DATA_BLOCK "PR"
TITLE =
VERSION : 0.1


  STRUCT
   rKmA_DlmHzl : INT ;	//EVS 100 HIZLI DOLUM % HIZ SET DEGERI
   rKmA_DlmYvs : INT ;	//EVS 100 YAVAS DOLUM % HIZ SET DEGERI
   rKmA_BsltHzl : INT ;	//EVS 100 HIZLI DOLUM % HIZ SET DEGERI
   rKmA_BsltYvs : INT ;	//EVS 100 YAVAS DOLUM % HIZ SET DEGERI
   rKmB_DlmHzl : INT ;	//EVS 100 HIZLI DOLUM % HIZ SET DEGERI
   rKmB_DlmYvs : INT ;	//EVS 100 YAVAS DOLUM % HIZ SET DEGERI
   rKmB_BsltHzl : INT ;	//EVS 100 HIZLI DOLUM % HIZ SET DEGERI
   rKmB_BsltYvs : INT ;	//EVS 100 YAVAS DOLUM % HIZ SET DEGERI
   rSd_BsltHzl : INT ;	//EVS 100 HIZLI DOLUM % HIZ SET DEGERI
   rSd_BsltYvs : INT ;	//EVS 100 YAVAS DOLUM % HIZ SET DEGERI
   rKl_BsltHzl : INT ;	//EVS 100 HIZLI DOLUM % HIZ SET DEGERI
   rKl_BsltYvs : INT ;	//EVS 100 YAVAS DOLUM % HIZ SET DEGERI
   rFl_BsltHzl : INT ;	//EVS 100 HIZLI DOLUM % HIZ SET DEGERI
   rFl_BsltYvs : INT ;	//EVS 100 YAVAS DOLUM % HIZ SET DEGERI
   rSl_BsltHzl : INT ;	//EVS 100 HIZLI DOLUM % HIZ SET DEGERI
   rSl_BsltYvs : INT ;	//EVS 100 YAVAS DOLUM % HIZ SET DEGERI
   rHm_BsltHzl : INT ;	//EVS 100 HIZLI DOLUM % HIZ SET DEGERI
   rHm_BsltYvs : INT ;	//EVS 100 YAVAS DOLUM % HIZ SET DEGERI
   rAn_BsltHzl : INT ;	//EVS 100 HIZLI DOLUM % HIZ SET DEGERI
   rAn_BsltYvs : INT ;	//EVS 100 YAVAS DOLUM % HIZ SET DEGERI
   YD : INT ;
   YD1 : INT ;
   YD2 : INT ;
   YD3 : INT ;
   YD4 : INT ;
   wKmA_DlmHzl { S7_m_c := 'true' }: INT ;	//EVS 100 HIZLI DOLUM % HIZ SET DEGERI
   wKmA_DlmYvs { S7_m_c := 'true' }: INT ;	//EVS 100 YAVAS DOLUM % HIZ SET DEGERI
   wKmA_BsltHzl { S7_m_c := 'true' }: INT ;	//EVS 100 HIZLI DOLUM % HIZ SET DEGERI
   wKmA_BsltYvs { S7_m_c := 'true' }: INT ;	//EVS 100 YAVAS DOLUM % HIZ SET DEGERI
   wKmB_DlmHzl { S7_m_c := 'true' }: INT ;	//EVS 100 HIZLI DOLUM % HIZ SET DEGERI
   wKmB_DlmYvs { S7_m_c := 'true' }: INT ;	//EVS 100 YAVAS DOLUM % HIZ SET DEGERI
   wKmB_BsltHzl { S7_m_c := 'true' }: INT ;	//EVS 100 HIZLI DOLUM % HIZ SET DEGERI
   wKmB_BsltYvs { S7_m_c := 'true' }: INT ;	//EVS 100 YAVAS DOLUM % HIZ SET DEGERI
   wSd_BsltHzl { S7_m_c := 'true' }: INT ;	//EVS 100 HIZLI DOLUM % HIZ SET DEGERI
   wSd_BsltYvs { S7_m_c := 'true' }: INT ;	//EVS 100 YAVAS DOLUM % HIZ SET DEGERI
   wKl_BsltHzl { S7_m_c := 'true' }: INT ;	//EVS 100 HIZLI DOLUM % HIZ SET DEGERI
   wKl_BsltYvs { S7_m_c := 'true' }: INT ;	//EVS 100 YAVAS DOLUM % HIZ SET DEGERI
   wFl_BsltHzl { S7_m_c := 'true' }: INT ;	//EVS 100 HIZLI DOLUM % HIZ SET DEGERI
   wFl_BsltYvs { S7_m_c := 'true' }: INT ;	//EVS 100 YAVAS DOLUM % HIZ SET DEGERI
   wSl_BsltHzl { S7_m_c := 'true' }: INT ;	//EVS 100 HIZLI DOLUM % HIZ SET DEGERI
   wSl_BsltYvs { S7_m_c := 'true' }: INT ;	//EVS 100 YAVAS DOLUM % HIZ SET DEGERI
   wHm_BsltHzl { S7_m_c := 'true' }: INT ;	//EVS 100 HIZLI DOLUM % HIZ SET DEGERI
   wHm_BsltYvs { S7_m_c := 'true' }: INT ;	//EVS 100 YAVAS DOLUM % HIZ SET DEGERI
   wAn_BsltHzl { S7_m_c := 'true' }: INT ;	//EVS 100 HIZLI DOLUM % HIZ SET DEGERI
   wAn_BsltYvs { S7_m_c := 'true' }: INT ;	//EVS 100 YAVAS DOLUM % HIZ SET DEGERI
   YD5 : INT ;
   KmANEM_ORAN { S7_m_c := 'true' }: REAL ;	//NEM ORAN
   KmBNEM_ORAN { S7_m_c := 'true' }: REAL ;	//NEM ORAN
   SdNEM_ORAN { S7_m_c := 'true' }: REAL ;	//NEM ORAN
   DlNEM_ORAN { S7_m_c := 'true' }: REAL ;	//NEM ORAN
   KlNEM_ORAN { S7_m_c := 'true' }: REAL ;	//NEM ORAN
   FlNEM_ORAN { S7_m_c := 'true' }: REAL ;	//NEM ORAN
   SlNEM_ORAN { S7_m_c := 'true' }: REAL ;	//NEM ORAN
   HmNEM_ORAN { S7_m_c := 'true' }: REAL ;	//NEM ORAN
   AnNEM_ORAN { S7_m_c := 'true' }: REAL ;	//NEM ORAN
   Renk1NEM_ORAN : REAL ;	//NEM ORAN
   Renk2NEM_ORAN : REAL ;	//NEM ORAN
   Renk3NEM_ORAN : REAL ;	//NEM ORAN
   Renk4NEM_ORAN : REAL ;	//NEM ORAN
   KmA_TolKg { S7_m_c := 'true' }: REAL ;	//DOZAJ TOLARANS KG
   KmB_TolKg { S7_m_c := 'true' }: REAL ;	//DOZAJ TOLARANS KG
   Sd_TolKg { S7_m_c := 'true' }: REAL ;	//DOZAJ TOLARANS KG
   Dl_TolKg { S7_m_c := 'true' }: REAL ;	//DOZAJ TOLARANS KG
   Kl_TolKg { S7_m_c := 'true' }: REAL ;	//DOZAJ TOLARANS KG
   Fl_TolKg { S7_m_c := 'true' }: REAL ;	//DOZAJ TOLARANS KG
   Sl_TolKg { S7_m_c := 'true' }: REAL ;	//DOZAJ TOLARANS KG
   Hm_TolKg { S7_m_c := 'true' }: REAL ;	//DOZAJ TOLARANS KG
   An_TolKg { S7_m_c := 'true' }: REAL ;	//DOZAJ TOLARANS KG
   Renk1_TolKg : REAL ;	//DOZAJ TOLARANS KG
   Renk2_TolKg : REAL ;	//DOZAJ TOLARANS KG
   Renk3_TolKg : REAL ;	//DOZAJ TOLARANS KG
   Renk4_TolKg : REAL ;	//DOZAJ TOLARANS KG
  END_STRUCT ;
BEGIN
   rKmA_DlmHzl := 0;
   rKmA_DlmYvs := 90;
   rKmA_BsltHzl := 65;
   rKmA_BsltYvs := 48;
   rKmB_DlmHzl := 0;
   rKmB_DlmYvs := 70;
   rKmB_BsltHzl := 60;
   rKmB_BsltYvs := 35;
   rSd_BsltHzl := 60;
   rSd_BsltYvs := 55;
   rKl_BsltHzl := 85;
   rKl_BsltYvs := 70;
   rFl_BsltHzl := 60;
   rFl_BsltYvs := 50;
   rSl_BsltHzl := 40;
   rSl_BsltYvs := 25;
   rHm_BsltHzl := 70;
   rHm_BsltYvs := 60;
   rAn_BsltHzl := 0;
   rAn_BsltYvs := 0;
   YD := 0;
   YD1 := 0;
   YD2 := 0;
   YD3 := 0;
   YD4 := 0;
   wKmA_DlmHzl := 0;
   wKmA_DlmYvs := 90;
   wKmA_BsltHzl := 65;
   wKmA_BsltYvs := 48;
   wKmB_DlmHzl := 0;
   wKmB_DlmYvs := 70;
   wKmB_BsltHzl := 60;
   wKmB_BsltYvs := 35;
   wSd_BsltHzl := 60;
   wSd_BsltYvs := 55;
   wKl_BsltHzl := 85;
   wKl_BsltYvs := 70;
   wFl_BsltHzl := 60;
   wFl_BsltYvs := 50;
   wSl_BsltHzl := 40;
   wSl_BsltYvs := 25;
   wHm_BsltHzl := 70;
   wHm_BsltYvs := 60;
   wAn_BsltHzl := 0;
   wAn_BsltYvs := 0;
   YD5 := 0;
   KmANEM_ORAN := 0.000000e+000;
   KmBNEM_ORAN := 0.000000e+000;
   SdNEM_ORAN := 0.000000e+000;
   DlNEM_ORAN := 0.000000e+000;
   KlNEM_ORAN := 0.000000e+000;
   FlNEM_ORAN := 0.000000e+000;
   SlNEM_ORAN := 0.000000e+000;
   HmNEM_ORAN := 0.000000e+000;
   AnNEM_ORAN := 0.000000e+000;
   Renk1NEM_ORAN := 0.000000e+000;
   Renk2NEM_ORAN := 0.000000e+000;
   Renk3NEM_ORAN := 0.000000e+000;
   Renk4NEM_ORAN := 0.000000e+000;
   KmA_TolKg := 0.000000e+000;
   KmB_TolKg := 0.000000e+000;
   Sd_TolKg := 0.000000e+000;
   Dl_TolKg := 0.000000e+000;
   Kl_TolKg := 0.000000e+000;
   Fl_TolKg := 0.000000e+000;
   Sl_TolKg := 0.000000e+000;
   Hm_TolKg := 0.000000e+000;
   An_TolKg := 0.000000e+000;
   Renk1_TolKg := 0.000000e+000;
   Renk2_TolKg := 0.000000e+000;
   Renk3_TolKg := 0.000000e+000;
   Renk4_TolKg := 0.000000e+000;
END_DATA_BLOCK

